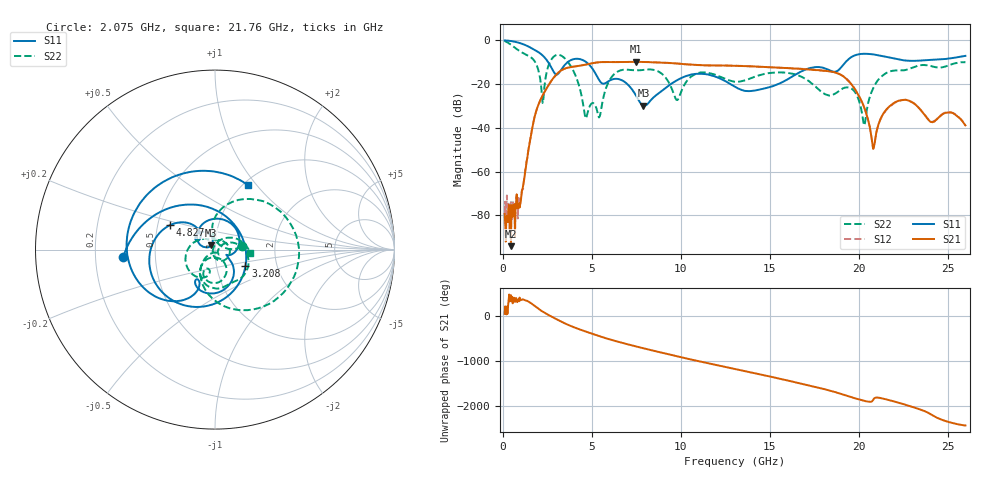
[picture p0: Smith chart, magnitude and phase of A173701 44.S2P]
!  2-Port S-parameters saved by WinCal
! VAR MeasName=S-Parameters (CALIBRATED_DATA) read from VNA (N5245A)
! VAR MeasDate=2017-6-7 10:31:20
! VAR NAME=A173701 44
! VAR FILENAME=A173701 44.S2P
! VAR DATE=2017-6-7 10:31:20
! VAR PHYS_PORTS=1,2
# Hz S DB R 50
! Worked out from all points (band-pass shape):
!   801 points, 100 MHz to 26 GHz, reference 50 ohm
!   highest |S21| = -9.78 dB at 7.481 GHz (marker M1); lowest = -94.0 dB at 456.1 MHz (marker M2)
!   |S21| within 3 dB of the highest: 3.521 GHz to 16.25 GHz (12.73 GHz wide, 129 % of centre)
!   lowest |S11| = -29.9 dB at 7.902 GHz (marker M3), VSWR 1.07, Z = 47.8 + j2.27 ohm
!   |S11| at or under -10 dB: 2.554 GHz to 3.635 GHz (1.081 GHz wide, 34.9 % of centre); 4.703 GHz to 19.26 GHz (14.55 GHz wide, 121 % of centre)
!   |S22| runs from -38.8 to -0.2 dB; largest |S21 - S12| = 0.0051
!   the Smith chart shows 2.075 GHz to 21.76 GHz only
!   S11 on the Smith chart (normalised r, x): 2.075 GHz: 0.32, -0.04; 3.208 GHz: 1.38, -0.27; 4.827 GHz: 0.58, +0.17; 21.76 GHz: 1.05, +0.90
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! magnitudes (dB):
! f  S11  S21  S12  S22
! 100 MHz  0.0  -79.3  -83.9  -0.2
! 456.1 MHz  -0.3  -94.0  -73.8  -1.9
! 974.1 MHz  -1.3  -75.0  -72.9  -5.0
! 2.075 GHz  -5.8  -27.9  -27.9  -16.4
! 2.269 GHz  -7.1  -24.6  -24.6  -27.7
! 3.208 GHz  -14.3  -14.1  -14.1  -6.7
! 4.438 GHz  -8.8  -11.4  -11.4  -25.9
! 4.827 GHz  -10.9  -10.8  -10.8  -31.3
! 6.316 GHz  -17.5  -9.9  -9.9  -15.0
! 7.481 GHz  -25.1  -9.8  -9.8  -13.7
! 7.902 GHz  -29.9  -9.9  -9.9  -13.5
! 8.744 GHz  -24.2  -10.1  -10.1  -14.2
! 9.78 GHz  -18.2  -10.5  -10.6  -27.3
! 10.98 GHz  -15.2  -11.2  -11.3  -14.9
! 13.05 GHz  -21.2  -11.6  -11.6  -18.9
! 17.39 GHz  -12.4  -13.4  -13.3  -19.8
! 19.62 GHz  -7.5  -20.4  -20.3  -22.2
! 20.3 GHz  -6.1  -30.4  -30.5  -38.8
! 20.85 GHz  -6.4  -48.9  -48.8  -21.3
! 21.69 GHz  -7.8  -30.4  -30.6  -14.3
! 21.76 GHz  -7.9  -30.0  -30.2  -14.2
! 26 GHz  -7.1  -38.8  -38.8  -10.0
